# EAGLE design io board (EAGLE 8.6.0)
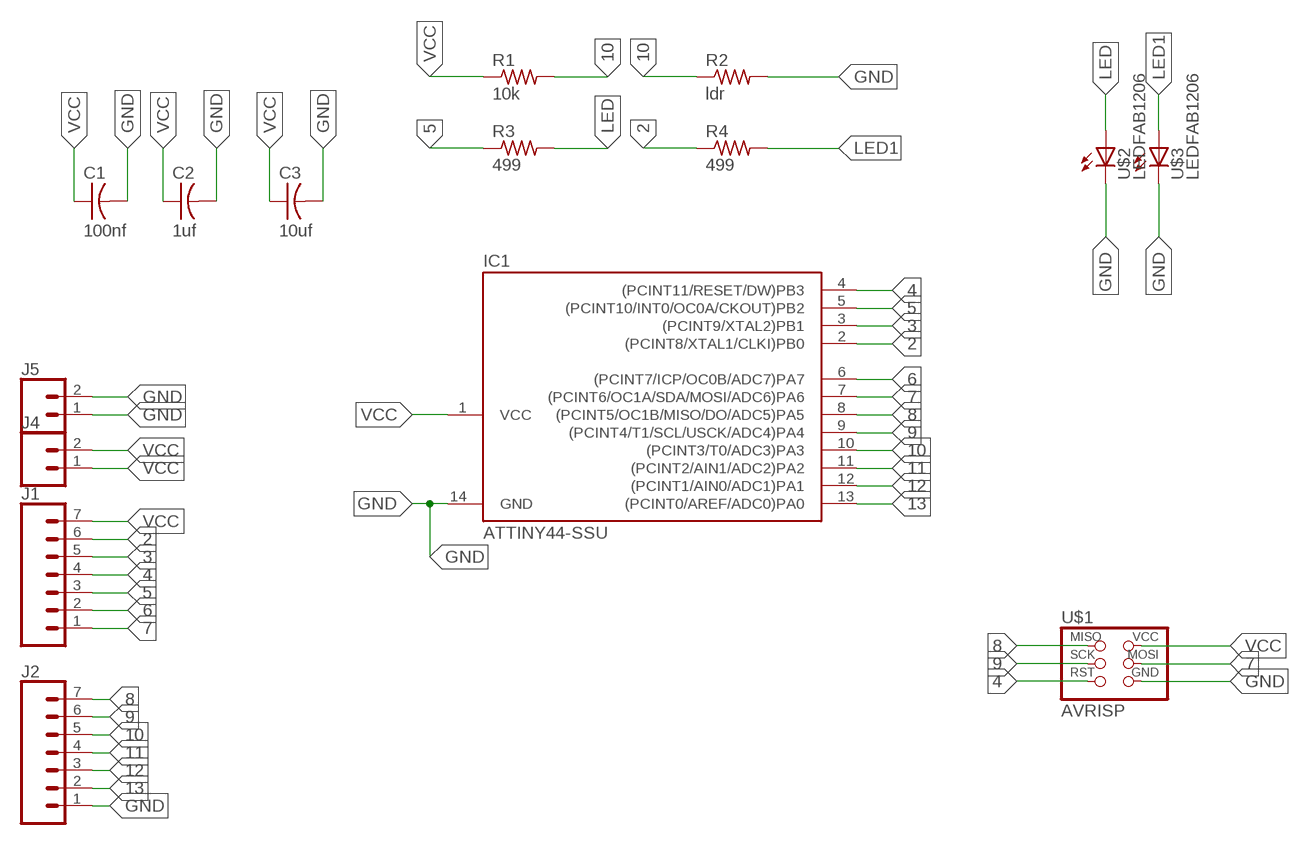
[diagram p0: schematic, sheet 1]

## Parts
C1  100nf  CAP-US1206FAB  [C1206FAB]
C2  1uf  CAP-US1206FAB  [C1206FAB]
C3  10uf  CAP-US1206FAB  [C1206FAB]
IC1  ATTINY44-SSU  [SOIC14]
J1  CONN_07  [1X07]
J2  CONN_07  [1X07]
J4  CONN_02  [1X02]
J5  CONN_02  [1X02]
R1  10k  RES-US1206FAB  [R1206FAB]
R2  ldr  RES-US1206FAB  [R1206FAB]
R3  499  RES-US1206FAB  [R1206FAB]
R4  499  RES-US1206FAB  [R1206FAB]
U$1  AVRISP  [2X03]
U$2  LEDFAB1206  [LED1206FAB]
U$3  LEDFAB1206  [LED1206FAB]

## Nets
2: IC1.2((PCINT8/XTAL1/CLKI)PB0) J1.6 R4.1
3: IC1.3((PCINT9/XTAL2)PB1) J1.5
4: IC1.4((PCINT11/RESET/DW)PB3) J1.4 U$1.5(RST)
5: IC1.5((PCINT10/INT0/OC0A/CKOUT)PB2) J1.3 R3.1
6: IC1.6((PCINT7/ICP/OC0B/ADC7)PA7) J1.2
7: IC1.7((PCINT6/OC1A/SDA/MOSI/ADC6)PA6) J1.1 U$1.4(MOSI)
8: IC1.8((PCINT5/OC1B/MISO/DO/ADC5)PA5) J2.7 U$1.1(MISO)
9: IC1.9((PCINT4/T1/SCL/USCK/ADC4)PA4) J2.6 U$1.3(SCK)
10: IC1.10((PCINT3/T0/ADC3)PA3) J2.5 R1.2 R2.1
11: IC1.11((PCINT2/AIN1/ADC2)PA2) J2.4
12: IC1.12((PCINT1/AIN0/ADC1)PA1) J2.3
13: IC1.13((PCINT0/AREF/ADC0)PA0) J2.2
GND: C1.2 C2.2 C3.2 IC1.14(GND) J2.1 J5.1 J5.2 R2.2 U$1.6(GND) U$2.2(C) U$3.2(C)
LED: R3.2 U$2.1(A)
LED1: R4.2 U$3.1(A)
VCC: C1.1 C2.1 C3.1 IC1.1(VCC) J1.7 J4.1 J4.2 R1.1 U$1.2(VCC)

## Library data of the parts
C1 = fab:CAP-US; MF: MULTICOMP; MPN: MC0805Y104M500A2.54MM; OC_FARNELL: 2112751
C2 C3 = fab:CAP-US; OC_FARNELL: unknown
IC1 = fab:ATTINY44; OC_FARNELL: unknown
J1 J2 = SparkFun-Connectors:CONN_07: Multi connection point. Often used as Generic Header-pin footprint for 0.1 inch spaced/style header connections On any of the 0.1 inch spaced packages, you can populate with these: Break Away Headers - Straight (PRT-00116) Break Away Male Headers - Right Angle (PRT-00553) Female Headers (PRT-00115)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; OC_FARNELL: unknown
J4 J5 = SparkFun-Connectors:CONN_02: Multi connection point. Often used as Generic Header-pin footprint for 0.1 inch spaced/style header connections; OC_FARNELL: unknown
R1-R4 = fab:RES-US: Resistor (US Symbol); OC_FARNELL: unknown
U$1 = fab:AVRISP; OC_FARNELL: unknown
U$2 U$3 = fab:LED: LED; OC_FARNELL: unknown

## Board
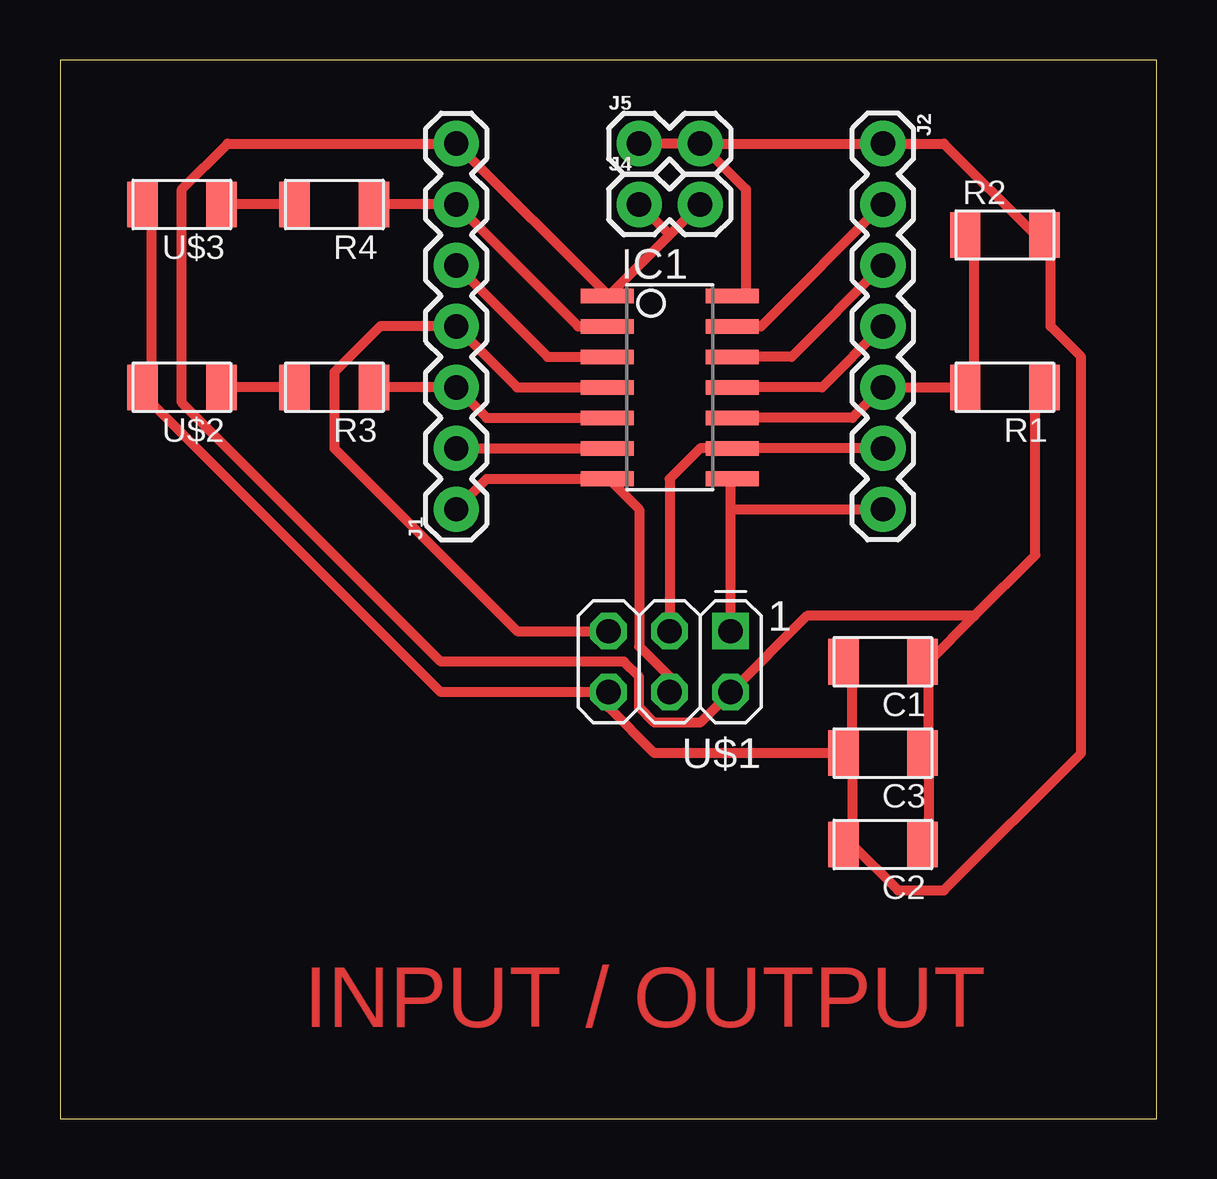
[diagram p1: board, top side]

Size 45.7 x 44.12 mm. Coordinates in mm from the lower left corner, seen from the top.
Outline: 0,0 45.7,0 45.7,44.12 0,44.12 0,0
Copper layers (1*16): Top 0.035mm / dielectric 1.5mm / Bottom 0.035mm
Design rules "default *": minimum track width 16mil, minimum drill 0.35mm, track to track 10mil, track to pad 10mil, pad to pad 10mil, via to via 10mil, smd to smd 10mil, copper to edge 40mil, drill to drill 6mil, minimum pad ring 10mil, minimum via ring 8mil, stop-mask expansion 4mil, vias tented up to drill 0mil, thermal gap 10mil

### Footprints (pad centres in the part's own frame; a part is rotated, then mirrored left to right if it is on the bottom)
C1206FAB = smd 1.27 x 1.905: 1 -1.651,0; 2 1.651,0
SOIC14 = smd 0.61 x 2.21: 1 -3.81,-2.603; 2 -2.54,-2.603; 3 -1.27,-2.603; 4 0,-2.603; 5 1.27,-2.603; 6 2.54,-2.603; 7 3.81,-2.603; 8 3.81,2.603; 9 2.54,2.603; 10 1.27,2.603; 11 0,2.603; 12 -1.27,2.603; 13 -2.54,2.603; 14 -3.81,2.603
1X07 = drill 1.016 pad 1.88: 1 0,0; 2 2.54,0; 3 5.08,0; 4 7.62,0; 5 10.16,0; 6 12.7,0; 7 15.24,0
1X02 = drill 1.016 pad 1.88: 1 0,0; 2 2.54,0
R1206FAB = smd 1.27 x 1.905: 1 -1.651,0; 2 1.651,0
2X03 = drill 1.016 square: 1 -2.54,-1.27 | drill 1.016 octagon: 2 -2.54,1.27; 3 0,-1.27; 4 0,1.27; 5 2.54,-1.27; 6 2.54,1.27
LED1206FAB = smd 1.27 x 1.905: 1 -1.651,0; 2 1.651,0

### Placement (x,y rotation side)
C1  34.29,19.05 180 top
C2  34.29,11.43 180 top
C3  34.29,15.24 180 top
IC1  25.4,30.48 270 top
J1  16.51,25.4 90 top
J2  34.29,40.64 270 top
J4  24.13,38.1 0 top
J5  24.13,40.64 0 top
R1  39.37,30.48 180 top
R2  39.37,36.83 0 top
R3  11.43,30.48 180 top
R4  11.43,38.1 180 top
U$1  25.4,19.05 180 top
U$2  5.08,30.48 180 top
U$3  5.08,38.1 180 top

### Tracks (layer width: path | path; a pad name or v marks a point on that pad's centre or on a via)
2
  Top 0.406: R4.1 J1.6 21.59,33.02 IC1.2
3
  Top 0.406: IC1.3 20.32,31.75 J1.5
4
  Top 0.406: IC1.4 19.05,30.48 J1.4 13.33,33.02 11.43,31.11 11.43,27.94 19.05,20.32 U$1.5
5
  Top 0.406: R3.1 J1.3 17.78,29.21 IC1.5
6
  Top 0.406: J1.2 IC1.6
7
  Top 0.406: J1.1 17.78,26.67 IC1.7 22.86,26.67 24.13,25.4 24.13,19.68 25.4,18.42 U$1.4
8
  Top 0.406: U$1.1 27.94,25.4 | 27.94,25.4 27.94,26.67 IC1.8 | 27.94,25.4 J2.7
9
  Top 0.406: J2.6 IC1.9 26.67,27.94 25.4,26.67 U$1.3
10
  Top 0.406: R2.1 38.1,36.83 38.1,30.48 R1.2 J2.5 33.02,29.21 IC1.10
11
  Top 0.406: IC1.11 31.75,30.48 J2.4
12
  Top 0.406: IC1.12 30.48,31.75 J2.3
13
  Top 0.406: IC1.13 29.21,33.02 J2.2
GND
  Top 0.406: J5.2 28.57,38.73 28.57,34.29 IC1.14 | J5.2 J5.1 | J5.2 J2.1 36.83,40.64 40.64,36.83 R2.2 41.28,36.83 41.28,33.02 42.55,31.75 42.55,15.24 36.83,9.52 34.92,9.52 33.02,11.43 | 3.81,30.48 3.81,38.1 U$3.2 | 33.02,15.24 33.02,11.43 | 33.02,15.24 33.02,19.05 C1.2 | 33.02,15.24 C3.2 24.76,15.24 22.86,17.14 U$1.6 15.87,17.78 3.81,29.85 3.81,30.48 | 3.81,30.48 U$2.2 | 33.02,11.43 C2.2
LED
  Top 0.406: R3.2 U$2.1
LED1
  Top 0.406: R4.2 U$3.1
VCC
  Top 0.406: J4.2 25.4,36.83 | 25.4,36.83 22.86,34.29 | 25.4,36.83 J4.1 | 22.86,34.29 J1.7 6.98,40.64 5.08,38.73 5.08,29.85 15.87,19.05 23.5,19.05 24.13,18.42 24.13,17.14 24.76,16.51 26.67,16.51 U$1.2 31.11,20.96 38.1,20.96 | 22.86,34.29 IC1.1 | 36.2,15.24 36.2,11.43 C2.1 | 36.2,15.24 36.2,19.05 | 36.2,15.24 C3.1 | 36.2,19.05 38.1,20.96 | 38.1,20.96 40.64,23.5 40.64,30.48 R1.1 | 36.2,19.05 C1.1

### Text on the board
Top: INPUT / OUTPUT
